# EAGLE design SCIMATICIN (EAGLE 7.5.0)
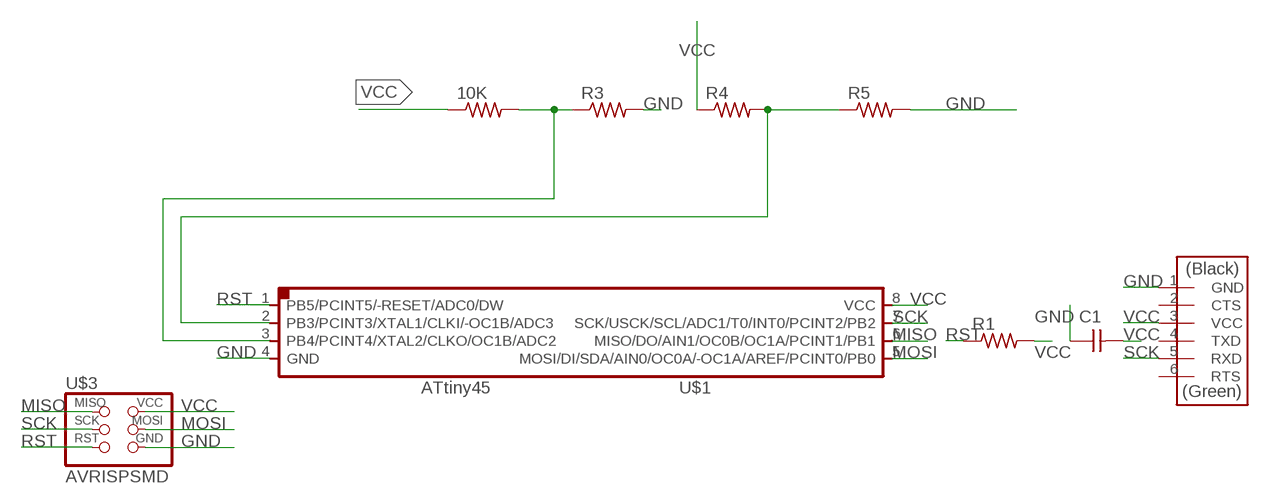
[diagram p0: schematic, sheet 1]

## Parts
10K  RES-US1206FAB  [R1206FAB]
C1  CAP-UNPOLARIZEDFAB  [C1206FAB]
R1  RES-US1206FAB  [R1206FAB]
R3  RES-US1206FAB  [R1206FAB]
R4  RES-US1206FAB  [R1206FAB]
R5  RES-US1206FAB  [R1206FAB]
U$1  ATTINY45SI  [SOIC8]
U$2  FTDI-SMD-HEADER  [1X06SMD]
U$3  AVRISPSMD  [2X03SMD]

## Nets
GND: C1.1 R3.2 R5.2 U$1.4(GND) U$2.1(GND) U$3.6(GND)
MISO: U$1.6(MISO/DO/AIN1/OC0B/OC1A/PCINT1/PB1) U$3.1(MISO)
MOSI: U$1.5(MOSI/DI/SDA/AIN0/OC0A/-OC1A/AREF/PCINT0/PB0) U$3.4(MOSI)
N$1: 10K.2 R3.1 U$1.3(PB4/PCINT4/XTAL2/CLKO/OC1B/ADC2)
N$2: R4.2 R5.1 U$1.2(PB3/PCINT3/XTAL1/CLKI/-OC1B/ADC3)
RST: R1.1 U$1.1(PB5/PCINT5/-RESET/ADC0/DW) U$3.5(RST)
SCK: U$1.7(SCK/USCK/SCL/ADC1/T0/INT0/PCINT2/PB2) U$2.5(RXD) U$3.3(SCK)
VCC: 10K.1 C1.2 R1.2 R4.1 U$1.8(VCC) U$2.3(VCC) U$3.2(VCC)
Unconnected: U$2.2(CTS) U$2.4(TXD) U$2.6(RTS)

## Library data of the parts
10K R1 R3-R5 = fab:RES-US: Resistor (US Symbol)
C1 = fab:CAP-UNPOLARIZED
U$1 = fab:ATTINY45
U$2 = fab:FTDI-SMD-HEADER
U$3 = fab:AVRISP

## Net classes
0 default: width 0.406 mm, drill 0.406 mm, clearance 0.406 mm

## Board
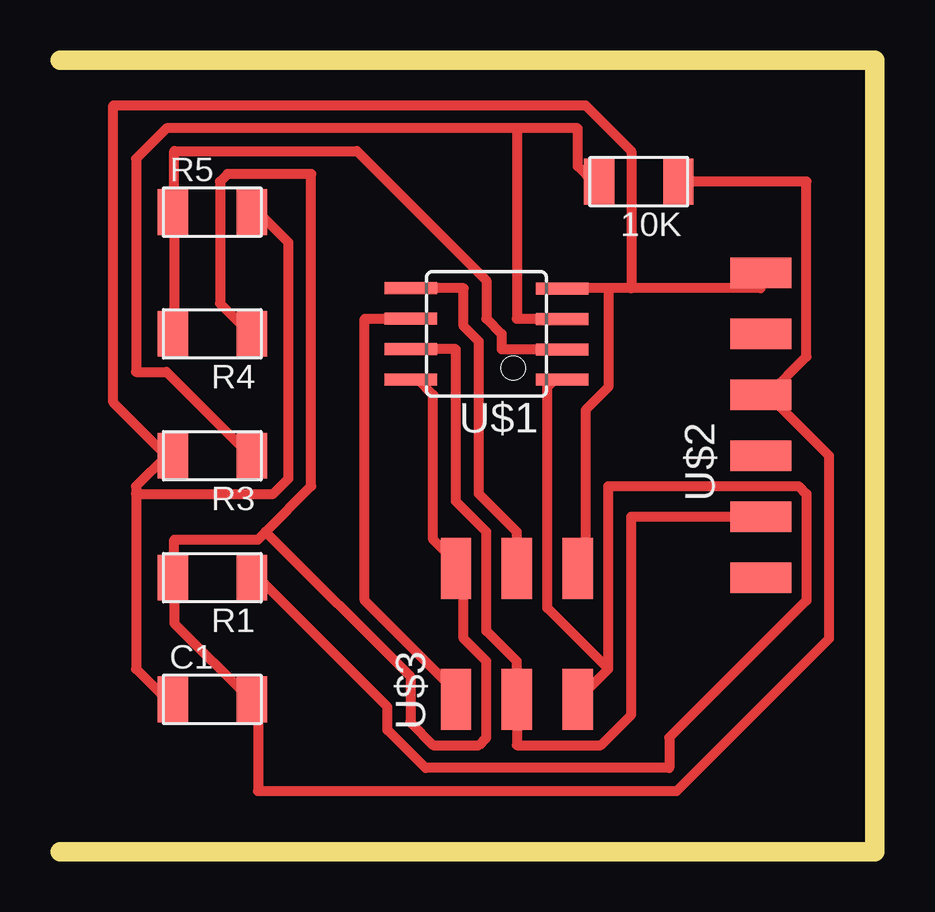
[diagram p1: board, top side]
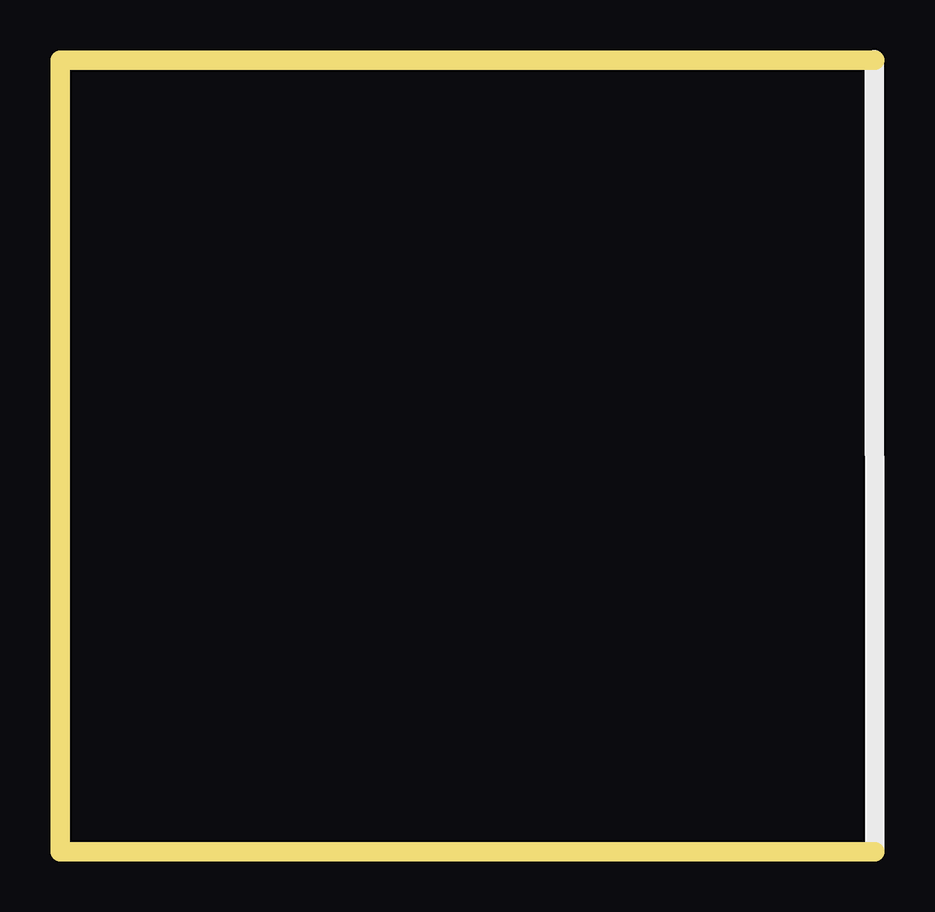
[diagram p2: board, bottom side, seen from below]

Size 33.96 x 33.01 mm. Coordinates in mm from the lower left corner, seen from the top.
Outline: 0,0 33.96,0 33.96,33.01 0,33.01
Copper layers (1*16): Top 0.035mm / dielectric 1.5mm / Bottom 0.035mm
Design rules "default *": minimum track width 10mil, minimum drill 24mil, track to track 16mil, track to pad 16mil, pad to pad 16mil, via to via 8mil, smd to smd 8mil, copper to edge 40mil, drill to drill 8mil, minimum pad ring 10mil, minimum via ring 8mil, stop-mask expansion 4mil, vias tented up to drill 0mil, thermal gap 10mil

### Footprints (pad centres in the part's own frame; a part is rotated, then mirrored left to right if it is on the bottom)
R1206FAB = smd 1.27 x 1.905: 1 -1.651,0; 2 1.651,0
C1206FAB = smd 1.27 x 1.905: 1 -1.651,0; 2 1.651,0
SOIC8 = smd 0.5 x 2.2: 1 -1.905,-3.154; 2 -0.645,-3.154; 3 0.625,-3.154; 4 1.895,-3.154; 5 1.905,3.154; 6 0.635,3.154; 7 -0.635,3.154; 8 -1.905,3.154
1X06SMD = smd 2.54 x 1.27: 1 0,6.35; 2 0,3.81; 3 0,1.27; 4 0,-1.27; 5 0,-3.81; 6 0,-6.35
2X03SMD = smd 2.54 x 1.27: 1 -2.54,2.54; 2 2.92,2.54; 3 -2.54,0; 4 2.92,0; 5 -2.54,-2.54; 6 2.92,-2.54

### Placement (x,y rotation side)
10K  24.13,27.94 180 top
C1  6.35,6.35 0 top
R1  6.35,11.43 180 top
R3  6.35,16.51 180 top
R4  6.35,21.59 180 top
R5  6.35,26.67 0 top
U$1  17.78,21.59 90 top
U$2  29.21,17.78 0 top
U$3  19.05,8.89 90 top

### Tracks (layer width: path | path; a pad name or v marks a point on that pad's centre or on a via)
GND
  Top 0.406: 23.81,23.49 29.21,23.49 U$2.1 | 23.81,23.49 22.86,23.49 | 22.86,23.49 20.96,23.49 U$1.4 | 22.86,23.49 22.86,19.37 21.91,18.41 21.91,12.38 21.59,12.06 U$3.6 | 3.18,14.92 3.18,15.24 4.45,16.51 | 3.18,14.92 3.18,7.62 4.45,6.35 C1.1 | 3.18,14.92 8.89,14.92 9.52,15.56 9.52,25.4 8.25,26.67 R5.2 | 23.81,23.49 23.81,29.21 21.91,31.11 2.22,31.11 2.22,18.73 4.45,16.51 | 4.45,16.51 R3.2
MISO
  Top 0.406: U$1.6 12.7,22.23 12.7,10.48 16.51,6.67 U$3.1
MOSI
  Top 0.406: U$1.5 16.83,23.49 16.83,21.91 17.46,21.27 17.46,14.92 19.05,13.33 U$3.4
N$1
  Top 0.406: 19.05,30.16 21.59,30.16 21.59,28.57 22.22,27.94 10K.2 | 19.05,30.16 4.45,30.16 3.18,28.89 3.18,20 4.45,20 7.94,16.51 R3.1 | 19.05,30.16 19.05,22.23 20.64,22.23 U$1.3
N$2
  Top 0.406: 4.76,26.67 4.76,21.59 R4.2 | 4.76,26.67 4.76,29.21 12.38,29.21 17.78,23.81 17.78,22.23 18.42,21.59 18.42,20.95 20.64,20.95 U$1.2 | 4.76,26.67 R5.1
RST
  Top 0.406: 22.86,7.62 22.86,15.24 30.8,15.24 31.11,14.92 31.11,10.48 25.4,4.76 25.4,3.49 15.24,3.49 13.65,5.08 13.65,6.03 8.25,11.43 R1.1 | U$3.5 22.86,7.62 | 22.86,7.62 20.32,10.16 20.32,19.37 20.64,19.68 U$1.1
SCK
  Top 0.406: U$1.7 16.51,20.95 16.51,14.6 17.78,13.33 17.78,9.21 19.05,7.94 U$3.3 19.05,4.44 22.54,4.44 23.81,5.71 23.81,13.97 U$2.5
VCC
  Top 0.406: 10K.1 31.11,27.94 31.11,20.64 29.53,19.05 | U$1.8 14.92,19.68 15.56,19.05 15.56,13.02 16.51,12.06 U$3.2 16.51,11.75 16.83,11.43 16.83,8.89 17.78,7.94 17.78,4.76 17.46,4.44 15.56,4.44 14.61,5.4 14.61,7.3 8.57,13.33 | 4.76,11.43 4.76,9.53 7.94,6.35 C1.2 8.25,6.35 8.25,2.54 25.72,2.54 32.07,8.89 32.07,16.51 29.53,19.05 | 8.57,13.33 8.25,13.02 4.76,13.02 4.76,11.43 | 8.57,13.33 10.48,15.24 10.48,28.26 6.98,28.26 6.67,27.94 6.67,22.86 7.94,21.59 R4.1 | 4.76,11.43 R1.2 | 29.53,19.05 U$2.3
